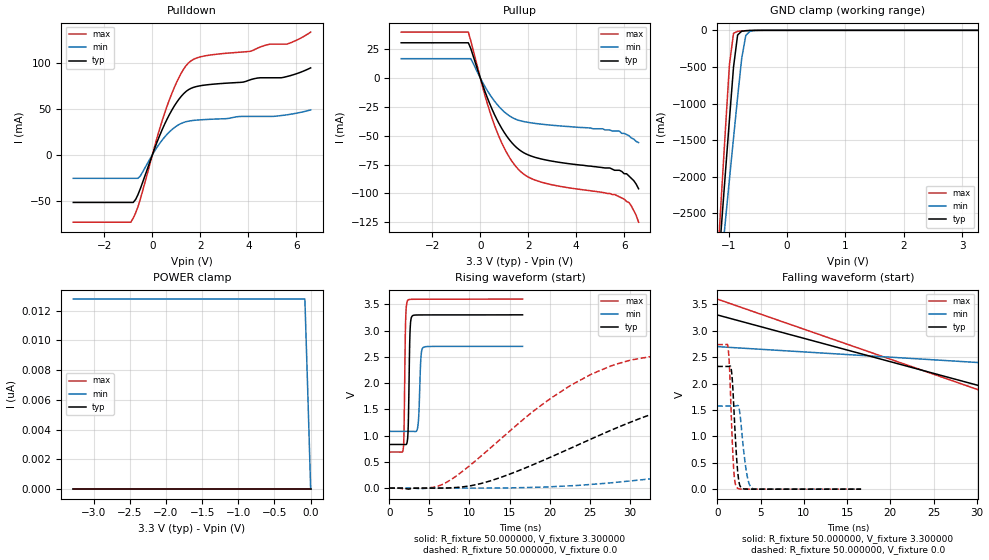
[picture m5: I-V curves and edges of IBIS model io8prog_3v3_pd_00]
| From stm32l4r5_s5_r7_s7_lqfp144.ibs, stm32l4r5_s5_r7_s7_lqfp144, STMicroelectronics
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|   Model io8prog_3v3_pd_00
[Model]  io8prog_3v3_pd_00
Model_type I/O
Polarity   Non-Inverting
Enable   Active-Low
Vinl =   0.990000V
Vinh =   2.310000V
Vmeas =  1.650000V
Cref =   100.000000nF
Rref =   1.000000k
Vref =   3.300000V
C_comp   2.267200pF   2.233100pF   2.322300pF
[Temperature Range]   25.000000   0.125000k   -40.000000
[Pullup Reference]   3.300000V   2.700000V   3.600000V
[Pulldown Reference]   0.0V   0.0V   0.0V
[POWER Clamp Reference]   3.300000V   2.700000V   3.600000V
[GND Clamp Reference]   0.0V   0.0V   0.0V
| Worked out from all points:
|   slope of the pulldown table from 0 to 0.495 V, typ, clamps not added: 15.3 ohm
|   slope of the pullup table from 0 to 0.495 V, typ, clamps not added: 18.1 ohm
|   GND clamp passes 1 mA (typ) near -0.58 V on its own axis
|   rising waveform, R_fixture 50.000000, V_fixture 3.300000: 20-80 % time 168ps typ, 221ps min, 156ps max; typ from 0.831 V to 3.3 V
|   rising waveform, R_fixture 50.000000, V_fixture 0.0: 20-80 % time 24.3ns typ, 54.5ns min, 14.6ns max; typ from 0 V to 2.32 V
|   falling waveform, R_fixture 50.000000, V_fixture 3.300000: 20-80 % time 33.4ns typ, 61.6ns min, 30.7ns max; typ from 3.3 V to 0.831 V
|   falling waveform, R_fixture 50.000000, V_fixture 0.0: 20-80 % time 474ps typ, 655ps min, 392ps max; typ from 2.32 V to 0 V
[Pulldown]
|Voltage   I(typ)   I(min)   I(max)
-3.3V     -51.86mA   -25.67mA   -73.32mA
-900mV    -51.86mA   -25.67mA   -73.32mA
-700mV    -48.68mA   -25.67mA   -63.27mA
-500mV    -36.68mA   -22.92mA   -47.9mA
200mV     14.09mA    8.363mA    18.97mA
700mV     43.2mA     24.54mA    59.15mA
1.2V      63.38mA    34mA       88.53mA
1.6V      72.01mA    36.89mA    101.8mA
4.1V      81.58mA    41.61mA    112.4mA
4.9V      83.61mA    41.61mA    120.1mA
5.6V      84.89mA    43.33mA    120.1mA
6.6V      94.39mA    48.68mA    133.3mA
[Pullup]
|Voltage   I(typ)   I(min)   I(max)
-3.3V     30.51mA    16.73mA    39.79mA
-500mV    30.51mA    16.73mA    39.79mA
-400mV    25.73mA    16.73mA    32.44mA
200mV     -11.99mA   -7.69mA    -15.6mA
500mV     -27.53mA   -17.49mA   -35.6mA
1V        -47.29mA   -29.38mA   -60.81mA
1.5V      -60.05mA   -35.95mA   -77.15mA
1.9V      -65.77mA   -38.13mA   -84.64mA
2.6V      -70.47mA   -40.14mA   -90.6mA
5.6V      -80mA      -46mA      -101mA
6.2V      -85mA      -50mA      -108mA
6.6V      -96mA      -56mA      -125mA
[GND_clamp]
|Voltage   I(typ)   I(min)   I(max)
-3.3V     -9.456A    -9.706A    -9.779A
-1.2V     -3.441A    -3.76A     -3.218A
-1.13V    -2.694A    -3.182A    -2.288A
-1.06V    -1.951A    -2.607A    -1.365A
-990mV    -1.216A    -2.035A    -464.9mA
-920mV    -500mA     -1.468A    -40.16mA
-850mV    -63.52mA   -913mA     -13.8mA
-780mV    -11.85mA   -384.3mA   -8.868mA
-710mV    -4.793mA   -70.28mA   -5.239mA
-640mV    -2.262mA   -14.31mA   -2.457mA
-430mV    -37.93uA   -161.8uA   -20.28uA
3.28V     87.11uA    89uA       71.58uA
[POWER_clamp]
|Voltage   I(typ)   I(min)   I(max)
-3.28V    0A         12.77nA    0A
-80mV     0A         12.77nA    0A
-40mV     0A         6.549nA    0A
0V        0A         0A         0A
[Ramp]
| variable   typ   min   max
dV/dt_r  1.39404/24.31899n   0.94416/54.54979n   1.64262/14.56547n
dV/dt_f  1.48081/21.07455n   0.97074/44.50667n   1.74729/13.65241n
R_load = 50.000000
[Rising Waveform]
R_fixture= 50.000000
V_fixture= 3.300000
V_fixture_min= 2.700000
V_fixture_max= 3.600000
|time   V(typ)   V(min)   V(max)
0s        830.9mV    1.081V     687.1mV
1.735ns   830.7mV    1.081V     744.7mV
1.835ns   830.4mV    1.081V     1.09V
2.035ns   828.4mV    1.081V     3.186V
2.302ns   979mV      1.081V     3.577V
2.569ns   2.917V     1.081V     3.593V
2.87ns    3.279V     1.08V      3.595V
3.57ns    3.296V     1.187V     3.596V
4.238ns   3.297V     2.679V     3.596V
16.62ns   3.299V     2.699V     3.599V
[Rising Waveform]
R_fixture= 50.000000
V_fixture= 0.0
V_fixture_min= 0.0
V_fixture_max= 0.0
|time   V(typ)   V(min)   V(max)
0s        2.475nV    39.58nV    2.334nV
7.207ns   2.236mV    -147.9uV   116.1mV
12.61ns   138.1mV    1.132mV    764.3mV
19.82ns   570.1mV    22.97mV    1.674V
27.63ns   1.1V       100.3mV    2.325V
41.44ns   1.814V     345.7mV    2.636V
64.26ns   2.213V     817.1mV    2.719V
88.29ns   2.289V     1.194V     2.735V
120.7ns   2.316V     1.444V     2.737V
299.1ns   2.323V     1.574V     2.738V
[Falling Waveform]
R_fixture= 50.000000
V_fixture= 3.300000
V_fixture_min= 2.700000
V_fixture_max= 3.600000
|time   V(typ)   V(min)   V(max)
0s        3.299V     2.699V     3.599V
50.05ns   1.083V     2.199V     749.3mV
100.1ns   858.2mV    1.294V     691.5mV
150.2ns   835.9mV    1.141V     687.6mV
200.2ns   831.9mV    1.101V     687.1mV
300.3ns   830.9mV    1.083V     687.1mV
4.955us   830.9mV    1.081V     687.1mV
[Falling Waveform]
R_fixture= 50.000000
V_fixture= 0.0
V_fixture_min= 0.0
V_fixture_max= 0.0
|time   V(typ)   V(min)   V(max)
0s        2.323V     1.574V     2.738V
1.235ns   2.323V     1.574V     2.704V
1.401ns   2.327V     1.574V     2.365V
1.602ns   2.291V     1.574V     1.498V
1.902ns   1.605V     1.574V     384.4mV
2.302ns   452.5mV    1.582V     24.09mV
2.703ns   40.64mV    1.312V     2.331mV
3.403ns   1.062mV    300.9mV    236.7uV
4.037ns   38.7uV     15.65mV    148.3uV
16.62ns   2.475nV    39.58nV    2.334nV
